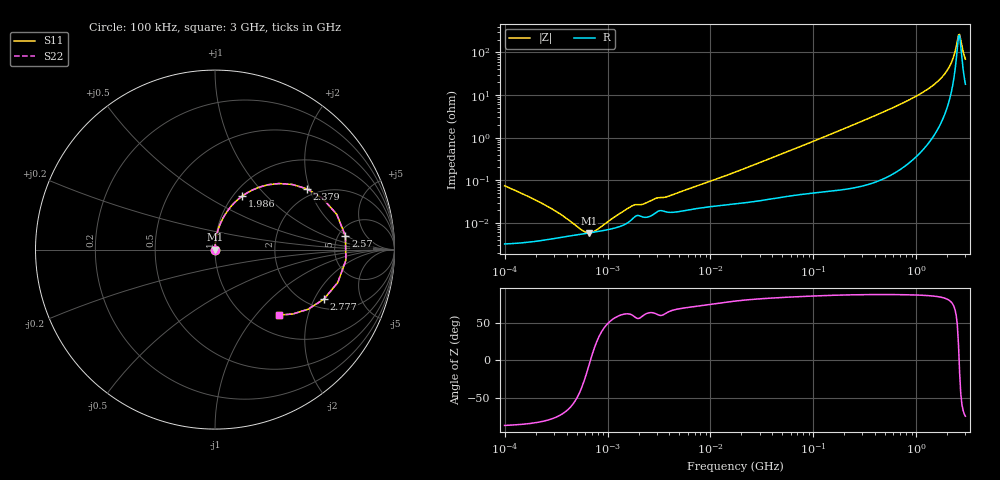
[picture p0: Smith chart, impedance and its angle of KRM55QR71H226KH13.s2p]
!Murata Part Number: KRM55QR71H226KH13
!These Parameters are Measured in Series Mode Connection
!Data Generated on Jan 08, 2026
!  o--ll--o
!Port1  Port2
!  o------o
!Operation Temp=25[degC], DC Bias Voltage=0[V]
!Freq. Start=100[kHz] Stop=3[GHz] 401[Steps]
# Hz S RI R 50
!Freq.(Hz) S11(Real) S11(Imag) S21(Real) S21(Imag) S12(Real) S12(Imag) S22(Real) S22(Imag)
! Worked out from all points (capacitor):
!   401 points, 100 kHz to 3 GHz, reference 50 ohm
!   read as one part in series: C = 21.1 uF near 105.3 kHz
!   lowest |Z| = 5.83 mohm at 656.3 kHz (marker M1)
!   series resonance near 681.7 kHz, so ESL is about 2.6 nH
!   S11 on the Smith chart (normalised r, x): 100 kHz: 1.00, -0.00; 1.986 GHz: 1.10, +0.74; 2.379 GHz: 1.77, +1.92; 2.57 GHz: 5.80, +1.88; 2.777 GHz: 2.42, -2.40; 3 GHz: 1.36, -1.34
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100000  3.26e-05 -0.000743  1 0.000743  1 0.000743  3.26e-05 -0.000743
240190  3.93e-05 -0.000269  1 0.000269  1 0.000269  3.93e-05 -0.000269
445844  5e-05 -9.16e-05  1 9.16e-05  1 9.16e-05  5e-05 -9.16e-05
562235  5.46e-05 -4.01e-05  0.9999 4.01e-05  0.9999 4.01e-05  5.46e-05 -4.01e-05
656258  5.78e-05 -7.8e-06  0.9999 7.8e-06  0.9999 7.8e-06  5.78e-05 -7.8e-06
965977  6.78e-05 7.24e-05  0.9999 -7.24e-05  0.9999 -7.24e-05  6.78e-05 7.24e-05
1747435  0.000124 0.00022  0.9999 -0.00022  0.9999 -0.00022  0.000124 0.00022
2203618  0.000137 0.000237  0.9999 -0.000237  0.9999 -0.000237  0.000137 0.000237
3161081  0.000191 0.000341  0.9998 -0.000341  0.9998 -0.000341  0.000191 0.000341
3986308  0.000177 0.000391  0.9998 -0.000391  0.9998 -0.000391  0.000177 0.000391
1.77727e7  0.000282 0.00156  0.9997 -0.00156  0.9997 -0.00156  0.000282 0.00156
9.738194e7  0.000561 0.00799  0.9994 -0.00799  0.9994 -0.00799  0.000561 0.00799
5.475153e8  0.00338 0.046  0.9966 -0.046  0.9966 -0.046  0.00338 0.046
1.24901e9  0.0226 0.1261  0.9774 -0.1261  0.9774 -0.1261  0.0226 0.1261
1.65839e9  0.0615 0.2037  0.9385 -0.2037  0.9385 -0.2037  0.0615 0.2037
1.986261e9  0.1519 0.2982  0.8481 -0.2982  0.8481 -0.2982  0.1519 0.2982
2.201951e9  0.2975 0.3616  0.7025 -0.3616  0.7025 -0.3616  0.2975 0.3616
2.378954e9  0.5131 0.3382  0.4869 -0.3382  0.4869 -0.3382  0.5131 0.3382
2.570185e9  0.7267 0.0757  0.2733 -0.0757  0.2733 -0.0757  0.7267 0.0757
2.637286e9  0.7291 -0.0592  0.2709 0.0592  0.2709 0.0592  0.7291 -0.0592
2.776789e9  0.6077 -0.2753  0.3923 0.2753  0.3923 0.2753  0.6077 -0.2753
3e9  0.3592 -0.3647  0.6408 0.3647  0.6408 0.3647  0.3592 -0.3647
